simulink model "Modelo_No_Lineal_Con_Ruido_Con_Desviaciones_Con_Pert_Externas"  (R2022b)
settings: Solver=ode4  StartTime=0.0  StopTime=0.2  FixedStep=1e-6  RelTol=1e-3
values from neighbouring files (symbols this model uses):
  C_DC = 6.8e-3    (= 0.0068)    [Sistema_no_lineal_Modal.m]    (also in Sistema_no_lineal_LQR.m; PI_Lazo_V_DC.m; LQR_Sin_Integral.m; LQR_Con_Integral.m)
  control = eye(2)    [Sistema_no_lineal_Modal.m]    (also in Sistema_no_lineal_LQR.m; Sistema_control_no_lineal_LQR.m; Sistema_control_no_lineal_Modal.m)
  eta_d0_1 = ((i_q0_1*omega_1 + v_d_1/L_1 - (R_1/L_1)*i_d0_1)*(2*m_t1*L_1))/V_DC0    [Sistema_no_lineal_Modal.m]    (also in Sistema_no_lineal_LQR.m; Sistema_control_no_lineal_LQR.m; Sistema_control_no_lineal_Modal.m)
  eta_d0_2 = ((i_q0_2*omega_2 + v_d_2/L_2 - (R_2/L_2)*i_d0_2)*(2*m_t2*L_2))/V_DC0    [Sistema_no_lineal_Modal.m]    (also in Sistema_no_lineal_LQR.m; Sistema_control_no_lineal_LQR.m; Sistema_control_no_lineal_Modal.m)
  eta_q0_1 = (- i_d0_1*omega_1 - (R_1/L_1)*i_q0_1)*(2*m_t1*L_1)/V_DC0    [Sistema_no_lineal_Modal.m]    (also in Sistema_no_lineal_LQR.m; Sistema_control_no_lineal_LQR.m; Sistema_control_no_lineal_Modal.m)
  eta_q0_2 = ((- i_d0_2*omega_2 - (R_2/L_2)*i_q0_2)*(2*m_t2*L_2))/V_DC0    [Sistema_no_lineal_Modal.m]    (also in Sistema_no_lineal_LQR.m; Sistema_control_no_lineal_LQR.m; Sistema_control_no_lineal_Modal.m)
  i_d0_1 = ((3000*2)/(3*v_d_1))*1.06522    [Sistema_no_lineal_Modal.m]    (also in Sistema_no_lineal_LQR.m; PI_Lazo_V_DC.m = 14.14213562; Sistema_control_no_lineal_LQR.m; Sistema_control_no_lineal_Modal.m)
  i_d0_2 = -i_d0_1/1.06522    [Sistema_no_lineal_Modal.m]    (also in Sistema_no_lineal_LQR.m; Sistema_control_no_lineal_LQR.m; Sistema_control_no_lineal_Modal.m)
  I_p_i_d_1 = 0.02    [Sistema_no_lineal_Modal.m]    (also in Sistema_no_lineal_LQR.m; Sistema_control_no_lineal_LQR.m = 0.2; Sistema_control_no_lineal_Modal.m = 0.2)
  I_p_i_d_2 = 0.02    [Sistema_no_lineal_Modal.m]    (also in Sistema_no_lineal_LQR.m; Sistema_control_no_lineal_LQR.m = 0.2; Sistema_control_no_lineal_Modal.m = 0.2)
  I_p_i_q_1 = 0.02    [Sistema_no_lineal_Modal.m]    (also in Sistema_no_lineal_LQR.m; Sistema_control_no_lineal_LQR.m = 0.2; Sistema_control_no_lineal_Modal.m = 0.2)
  i_q0_1 = 0    [Sistema_no_lineal_Modal.m]    (also in Sistema_no_lineal_LQR.m; Sistema_control_no_lineal_LQR.m; Sistema_control_no_lineal_Modal.m)
  i_q0_2 = 0    [Sistema_no_lineal_Modal.m]    (also in Sistema_no_lineal_LQR.m; Sistema_control_no_lineal_LQR.m; Sistema_control_no_lineal_Modal.m)
  Inst_Desv_C_DC = 0.1    [Sistema_no_lineal_Modal.m]    (also in Sistema_no_lineal_LQR.m; Sistema_control_no_lineal_LQR.m; Sistema_control_no_lineal_Modal.m)
  Inst_Desv_L_1 = 0.1    [Sistema_no_lineal_Modal.m]    (also in Sistema_no_lineal_LQR.m; Sistema_control_no_lineal_LQR.m; Sistema_control_no_lineal_Modal.m)
  Inst_Desv_L_2 = 0.1    [Sistema_no_lineal_Modal.m]    (also in Sistema_no_lineal_LQR.m; Sistema_control_no_lineal_LQR.m; Sistema_control_no_lineal_Modal.m)
  Inst_Desv_R_1 = 0.1    [Sistema_no_lineal_Modal.m]    (also in Sistema_no_lineal_LQR.m; Sistema_control_no_lineal_LQR.m; Sistema_control_no_lineal_Modal.m)
  Inst_Desv_R_2 = 0.1    [Sistema_no_lineal_Modal.m]    (also in Sistema_no_lineal_LQR.m; Sistema_control_no_lineal_LQR.m; Sistema_control_no_lineal_Modal.m)
  Kc1 = Kca_place1(:, 1:2)    [Sistema_no_lineal_Modal.m]    (also in Sistema_no_lineal_LQR.m = Kca1(:, 1:2); Sistema_control_no_lineal_LQR.m = Kca1(:, 1:2); Sistema_control_no_lineal_Modal.m)
  Kc2 = Kca_place2(:, 1:2)    [Sistema_no_lineal_Modal.m]    (also in Sistema_no_lineal_LQR.m = Kca2(:, 1:2); Sistema_control_no_lineal_LQR.m = Kca2(:, 1:2); Sistema_control_no_lineal_Modal.m)
  Ki1 = -Kca_place1(:, 3:4)    [Sistema_no_lineal_Modal.m]    (also in Sistema_no_lineal_LQR.m = -Kca1(:, 3:4); Sistema_control_no_lineal_LQR.m = -Kca1(:, 3:4); Sistema_control_no_lineal_Modal.m)
  Ki2 = -Kca_place2(:, 3:4)    [Sistema_no_lineal_Modal.m]    (also in Sistema_no_lineal_LQR.m = -Kca2(:, 3:4); Sistema_control_no_lineal_LQR.m = -Kca2(:, 3:4); Sistema_control_no_lineal_Modal.m)
  L_1 = 4.1e-3    (= 0.0041)    [Sistema_no_lineal_Modal.m]    (also in Sistema_no_lineal_LQR.m; Generadores_y_tranformadas.m; LQR_Sin_Integral.m; LQR_Con_Integral.m)
  L_2 = 5.3e-3    (= 0.0053)    [Sistema_no_lineal_Modal.m]    (also in Sistema_no_lineal_LQR.m; Generadores_y_tranformadas.m; Sistema_control_no_lineal_LQR.m; Sistema_control_no_lineal_Modal.m)
  m_t1 = 5    [Sistema_no_lineal_Modal.m]    (also in Sistema_no_lineal_LQR.m; LQR_Sin_Integral.m; LQR_Con_Integral.m; Modal_Integral.m)
  m_t2 = 5    [Sistema_no_lineal_Modal.m]    (also in Sistema_no_lineal_LQR.m; Sistema_control_no_lineal_LQR.m; Sistema_control_no_lineal_Modal.m)
  omega_1 = 377    [Sistema_no_lineal_Modal.m]    (also in Sistema_no_lineal_LQR.m; LQR_Sin_Integral.m; LQR_Con_Integral.m; Modal_Integral.m)
  omega_2 = 377    [Sistema_no_lineal_Modal.m]    (also in Sistema_no_lineal_LQR.m; Sistema_control_no_lineal_LQR.m; Sistema_control_no_lineal_Modal.m)
  p_i_d_1 = 1.5    [Sistema_no_lineal_Modal.m]    (also in Sistema_no_lineal_LQR.m; Sistema_control_no_lineal_LQR.m = 2.5; Sistema_control_no_lineal_Modal.m = 2.5)
  p_i_d_2 = 1.7    [Sistema_no_lineal_Modal.m]    (also in Sistema_no_lineal_LQR.m; Sistema_control_no_lineal_LQR.m = 2.7; Sistema_control_no_lineal_Modal.m = 2.7)
  p_i_q_1 = -1.3    [Sistema_no_lineal_Modal.m]    (also in Sistema_no_lineal_LQR.m; Sistema_control_no_lineal_LQR.m = -0.5; Sistema_control_no_lineal_Modal.m = -0.5)
  Porc_Desv_C_DC = 0.05    [Sistema_no_lineal_Modal.m]    (also in Sistema_no_lineal_LQR.m; Sistema_control_no_lineal_LQR.m; Sistema_control_no_lineal_Modal.m)
  Porc_Desv_L_1 = 0.05    [Sistema_no_lineal_Modal.m]    (also in Sistema_no_lineal_LQR.m; Sistema_control_no_lineal_LQR.m; Sistema_control_no_lineal_Modal.m)
  Porc_Desv_L_2 = 0.05    [Sistema_no_lineal_Modal.m]    (also in Sistema_no_lineal_LQR.m; Sistema_control_no_lineal_LQR.m; Sistema_control_no_lineal_Modal.m)
  Porc_Desv_R_1 = 0.05    [Sistema_no_lineal_Modal.m]    (also in Sistema_no_lineal_LQR.m; Sistema_control_no_lineal_LQR.m; Sistema_control_no_lineal_Modal.m)
  Porc_Desv_R_2 = 0.05    [Sistema_no_lineal_Modal.m]    (also in Sistema_no_lineal_LQR.m; Sistema_control_no_lineal_LQR.m; Sistema_control_no_lineal_Modal.m)
  R_1 = 284e-3    (= 0.284)    [Sistema_no_lineal_Modal.m]    (also in Sistema_no_lineal_LQR.m; Generadores_y_tranformadas.m; LQR_Sin_Integral.m; LQR_Con_Integral.m)
  R_2 = 330e-3    (= 0.33)    [Sistema_no_lineal_Modal.m]    (also in Sistema_no_lineal_LQR.m; Generadores_y_tranformadas.m; Sistema_control_no_lineal_LQR.m; Sistema_control_no_lineal_Modal.m)
  tau = te    (= 0.001)    [Sistema_no_lineal_Modal.m]    (also in Sistema_no_lineal_LQR.m; IP_Lazo_P_2.m = 0.002; IP_Lazo_Q_12.m = 0.002; LQR_Sin_Integral.m = 0.002)
  v_d_1 = 100*sqrt(2)    [Sistema_no_lineal_Modal.m]    (also in Sistema_no_lineal_LQR.m; PI_Lazo_V_DC.m; LQR_Sin_Integral.m; LQR_Con_Integral.m)
  v_d_2 = 100*sqrt(2)    [Sistema_no_lineal_Modal.m]    (also in Sistema_no_lineal_LQR.m; IP_Lazo_P_2.m; Sistema_control_no_lineal_LQR.m; Sistema_control_no_lineal_Modal.m)
  V_DC0 = 500    [Sistema_no_lineal_Modal.m]    (also in Sistema_no_lineal_LQR.m; PI_Lazo_V_DC.m; LQR_Sin_Integral.m; LQR_Con_Integral.m)
  V_R_i = D_R_i^2    (= 2.5e-05)    [Sistema_no_lineal_Modal.m]    (also in Sistema_no_lineal_LQR.m; LQR_Con_Integral.m; Modal_Integral.m; Sistema_control_no_lineal_LQR.m)
  V_R_V = D_R_V^2    (= 4e-06)    [Sistema_no_lineal_Modal.m]    (also in Sistema_no_lineal_LQR.m; PI_Lazo_V_DC.m = 0.0009; Sistema_control_no_lineal_LQR.m = 0.0009; Sistema_control_no_lineal_Modal.m = 0.0009)

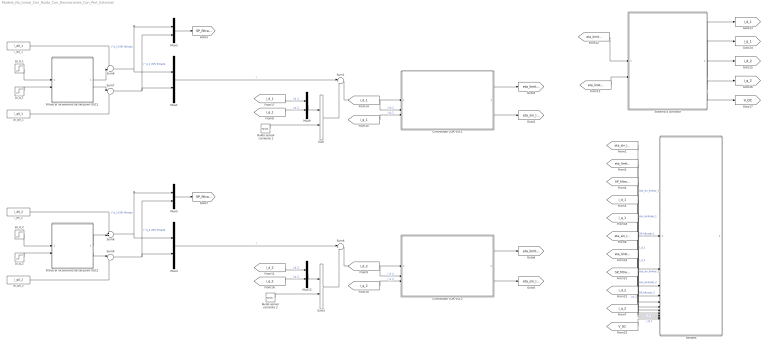
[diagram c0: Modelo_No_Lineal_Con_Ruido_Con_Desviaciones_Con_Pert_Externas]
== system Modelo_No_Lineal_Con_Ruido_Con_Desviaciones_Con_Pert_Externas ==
  Controlador LQR VSC1 : Subsystem
  Controlador LQR VSC2 : Subsystem
  Filtros al incremento de set-point VSC1 : Subsystem
  Filtros al incremento de set-point VSC2 : Subsystem
  Mux{1..2,4..5,9,12} (6 alike) : Mux  Inputs=2
  Ruido sensor corriente 1 : RandomNumber  Variance=V_R_i  SampleTime=0.001
  Ruido sensor corriente 2 : RandomNumber  Variance=V_R_i  SampleTime=0.001
  Señales : Subsystem
  Sistema a controlar : Subsystem
  Sum : Sum
  Sum1 : Sum  Inputs=|+-
  Sum2 : Sum
  Sum4 : Sum  Inputs=|+-
  Sum6 : Sum  Inputs=++|
  Sum7 : Sum  Inputs=|++
  Sum8 : Sum  Inputs=++|
  Sum9 : Sum  Inputs=|++
  i_d0_1 : Constant  Value=i_d0_1
  i_d0_2 : Constant  Value=i_d0_2
  Δi_d_1 : Step  Time=0.05  After=i_d0_1*0.05  SampleTime=0
  Δi_d_2 : Step  Time=0.05  After=i_d0_2*0.05  SampleTime=0
  Δi_q0_1 : Constant  Value=i_q0_1
  Δi_q0_2 : Constant  Value=i_q0_2
  Δi_q_1 : Step  Time=0.05  After=i_q0_1+0.5  SampleTime=0
  Δi_q_2 : Step  Time=0.05  After=i_q0_2-0.5  SampleTime=0
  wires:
  Mux2/1 -> [SP_filtrado_1]
  Δi_d_1/1 -> Filtros al incremento de set-point VSC1/1(Δi_d_1 sin filtrar)
  Δi_q_1/1 -> Filtros al incremento de set-point VSC1/2(Δi_q_1 sin filtrar)
  [eta_sin_limitar_1] -> Señales/1(eta_sin_limitar_1)  "eta_sin_limitar_1"
  [eta_limitado_1] -> Señales/2(eta_limitado_1)  "eta_limitado_1"
  [SP_filtrado_1] -> Señales/3(SP_filtrado_1)  "SP_filtrado_1"
  [i_d_1] -> Señales/4(i_d_1)  "i_d_1"
  Sum6/1 -> Mux2/1, Mux1/1  "i^d_1 (SP) filtrado"
  Sum7/1 -> Mux2/2, Mux1/2  "i^q_1 (SP) filtrado"
  Mux1/1 -> Sum1/1  "r"
  Sum9/1 -> Mux5/2, Mux4/2  "i^q_2 (SP) filtrado"
  Sum8/1 -> Mux4/1, Mux5/1  "i^d_2 (SP) filtrado"
  Mux5/1 -> [SP_filtrado_2]
  Sistema a controlar/1(i_d_1) -> [i_d_1]
  Sistema a controlar/2(i_q_1) -> [i_q_1]
  Sistema a controlar/3(i_d_2) -> [i_d_2]
  Sistema a controlar/4(i_q_2) -> [i_q_2]
  Sistema a controlar/5(V_DC) -> [V_DC]
  [eta_limitado_1] -> Sistema a controlar/1(eta limitado 1)
  [eta_limitado_2] -> Sistema a controlar/2(eta limitado 2)
  [i_d_1] -> Mux9/1  "i_d_2"
  [i_q_1] -> Mux9/2  "i_q_2"
  Mux9/1 -> Sum/1
  [i_q_1] -> Señales/5(i_q_1)  "i_q_1"
  [eta_sin_limitar_2] -> Señales/6(eta_sin_limitar_2)  "eta_sin_limitar_2"
  [eta_limitado_2] -> Señales/7(eta_limitado_2)  "eta_limitado_2"
  [SP_filtrado_2] -> Señales/8(SP_filtrado_2)  "SP_filtrado_2"
  [i_d_2] -> Señales/9(i_d_2)  "i_d_1"
  [i_q_2] -> Señales/10(i_q_2)  "i_q_1"
  [V_DC] -> Señales/11(V_DC)  "i_q_1"
  Mux12/1 -> Sum2/1
  [i_q_2] -> Mux12/2  "i_q_2"
  [i_d_2] -> Mux12/1  "i_d_2"
  Mux4/1 -> Sum4/1  "r"
  Filtros al incremento de set-point VSC1/1(Δi_d_1 filtrado) -> Sum6/2
  Filtros al incremento de set-point VSC1/2(Δi_q_1 filtrado) -> Sum7/1
  i_d0_1/1 -> Sum6/1
  Δi_q0_1/1 -> Sum7/2
  Δi_q0_2/1 -> Sum9/2
  i_d0_2/1 -> Sum8/1
  Filtros al incremento de set-point VSC2/2(Δi_q_2 filtrado) -> Sum9/1
  Filtros al incremento de set-point VSC2/1(Δi_d_2 filtrado) -> Sum8/2
  Δi_q_2/1 -> Filtros al incremento de set-point VSC2/2(Δi_q_2 sin filtrar)
  Δi_d_2/1 -> Filtros al incremento de set-point VSC2/1(Δi_d_2 sin filtrar)
  Sum1/1 -> Controlador LQR VSC1/1(e)
  [i_d_1] -> Controlador LQR VSC1/2(i_d_1)  "i_d_1"
  [i_q_1] -> Controlador LQR VSC1/3(i_q_1)  "i_q_1"
  Controlador LQR VSC1/1(eta limitado 1) -> [eta_limitado_1]
  Controlador LQR VSC1/2(eta sin limitar 1) -> [eta_sin_limitar_1]
  Sum4/1 -> Controlador LQR VSC2/1(e)
  [i_d_2] -> Controlador LQR VSC2/2(i_d_2)  "i_d_2"
  [i_q_2] -> Controlador LQR VSC2/3(i_q_2)  "i_q_2"
  Controlador LQR VSC2/1(eta limitado 2) -> [eta_limitado_2]
  Controlador LQR VSC2/2(eta sin limitar 2) -> [eta_sin_limitar_2]
  Ruido sensor corriente 1/1 -> Sum/2
  Ruido sensor corriente 2/1 -> Sum2/2
  Sum2/1 -> Sum4/2
  Sum/1 -> Sum1/2

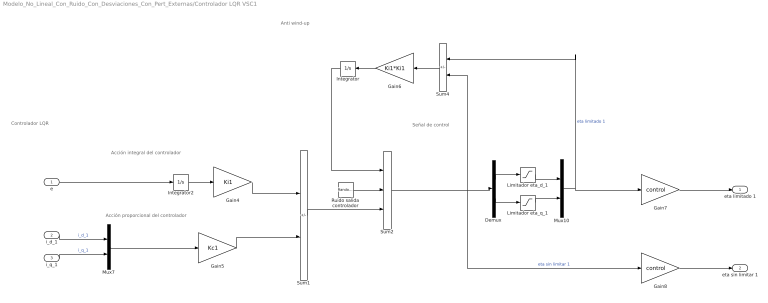
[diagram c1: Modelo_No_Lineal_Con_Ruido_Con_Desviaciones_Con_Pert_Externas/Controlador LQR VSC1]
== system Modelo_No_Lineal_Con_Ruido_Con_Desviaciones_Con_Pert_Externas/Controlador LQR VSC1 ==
  note: Anti wind-up
  note: Controlador LQR
  note: Acción proporcional del controlador
  note: Acción integral del controlador
  note: Señal de control
  e : Inport
  i_d_1 : Inport  Port=2
  i_q_1 : Inport  Port=3
  Demux : Demux  Outputs=2
  Gain4 : Gain  Gain=Ki1  Multiplication=Matrix(K*u) (u vector)
  Gain5 : Gain  Gain=Kc1  Multiplication=Matrix(K*u) (u vector)
  Gain6 : Gain  Gain=Ki1*Ki1  Multiplication=Matrix(K*u) (u vector)
  Gain7 : Gain  Gain=control  Multiplication=Matrix(K*u) (u vector)
  Gain8 : Gain  Gain=control  Multiplication=Matrix(K*u) (u vector)
  Integrator : Integrator
  Integrator2 : Integrator
  Limitador eta_d_1 : Saturate  UpperLimit=5 - eta_d0_1  LowerLimit=-5 - eta_d0_1
  Limitador eta_q_1 : Saturate  UpperLimit=5 - eta_q0_1  LowerLimit=-5 - eta_q0_1
  Mux10 : Mux  Inputs=2
  Mux7 : Mux  Inputs=2
  Ruido salida controlador : RandomNumber  Variance=V_R_V  SampleTime=0.001
  Sum1 : Sum  Inputs=+-
  Sum2 : Sum  Inputs=+++
  Sum4 : Sum  Inputs=+-
  eta limitado 1 : Outport
  eta sin limitar 1 : Outport  Port=2
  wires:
  i_q_1/1 -> Mux7/2  "i_q_1"
  Mux10/1 -> Sum4/1, Gain7/1  "eta limitado 1"
  Limitador eta_q_1/1 -> Mux10/2
  i_d_1/1 -> Mux7/1  "i_d_1"
  Limitador eta_d_1/1 -> Mux10/1
  Demux/2 -> Limitador eta_q_1/1
  Gain8/1 -> eta sin limitar 1/1
  Sum2/1 -> Gain8/1, Demux/1, Sum4/2  "eta sin limitar 1"
  Gain7/1 -> eta limitado 1/1
  Demux/1 -> Limitador eta_d_1/1
  Gain5/1 -> Sum1/2
  Gain4/1 -> Sum1/1
  Sum4/1 -> Gain6/1
  Mux7/1 -> Gain5/1
  Gain6/1 -> Integrator/1
  Sum1/1 -> Sum2/3
  Integrator2/1 -> Gain4/1
  e/1 -> Integrator2/1
  Integrator/1 -> Sum2/1
  Ruido salida controlador/1 -> Sum2/2

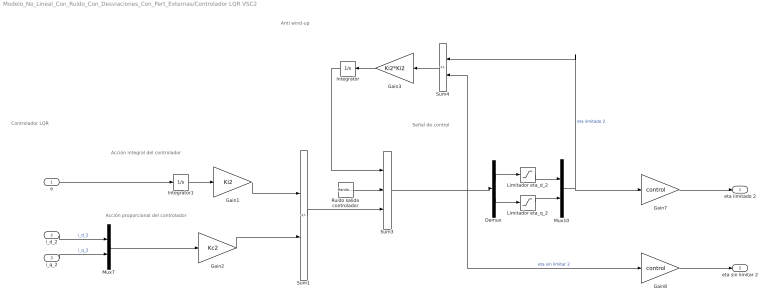
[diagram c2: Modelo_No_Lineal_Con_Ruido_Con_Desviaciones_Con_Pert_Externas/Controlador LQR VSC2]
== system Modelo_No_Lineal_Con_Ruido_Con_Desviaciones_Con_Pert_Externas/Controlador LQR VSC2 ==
  note: Señal de control
  note: Anti wind-up
  note: Acción proporcional del controlador
  note: Controlador LQR
  note: Acción integral del controlador
  e : Inport
  i_d_2 : Inport  Port=2
  i_q_2 : Inport  Port=3
  Demux : Demux  Outputs=2
  Gain1 : Gain  Gain=Ki2  Multiplication=Matrix(K*u) (u vector)
  Gain2 : Gain  Gain=Kc2  Multiplication=Matrix(K*u) (u vector)
  Gain3 : Gain  Gain=Ki2*Ki2  Multiplication=Matrix(K*u) (u vector)
  Gain7 : Gain  Gain=control  Multiplication=Matrix(K*u) (u vector)
  Gain8 : Gain  Gain=control  Multiplication=Matrix(K*u) (u vector)
  Integrator : Integrator
  Integrator1 : Integrator
  Limitador eta_d_2 : Saturate  UpperLimit=5 - eta_d0_2  LowerLimit=-5 - eta_d0_2
  Limitador eta_q_2 : Saturate  UpperLimit=5 - eta_q0_2  LowerLimit=-5 - eta_q0_2
  Mux10 : Mux  Inputs=2
  Mux7 : Mux  Inputs=2
  Ruido salida controlador : RandomNumber  Variance=V_R_V  SampleTime=0.001
  Sum1 : Sum  Inputs=+-
  Sum3 : Sum  Inputs=+++
  Sum4 : Sum  Inputs=+-
  eta limitado 2 : Outport
  eta sin limitar 2 : Outport  Port=2
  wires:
  Gain8/1 -> eta sin limitar 2/1
  Integrator/1 -> Sum3/1
  Mux7/1 -> Gain2/1
  i_d_2/1 -> Mux7/1  "i_d_2"
  Mux10/1 -> Sum4/1, Gain7/1  "eta limitado 2"
  Gain7/1 -> eta limitado 2/1
  Sum3/1 -> Gain8/1, Demux/1, Sum4/2  "eta sin limitar 2"
  i_q_2/1 -> Mux7/2  "i_q_2"
  Limitador eta_d_2/1 -> Mux10/1
  Limitador eta_q_2/1 -> Mux10/2
  Integrator1/1 -> Gain1/1
  Demux/2 -> Limitador eta_q_2/1
  Demux/1 -> Limitador eta_d_2/1
  Sum4/1 -> Gain3/1
  Gain3/1 -> Integrator/1
  Sum1/1 -> Sum3/3
  Gain1/1 -> Sum1/1
  Gain2/1 -> Sum1/2
  e/1 -> Integrator1/1
  Ruido salida controlador/1 -> Sum3/2

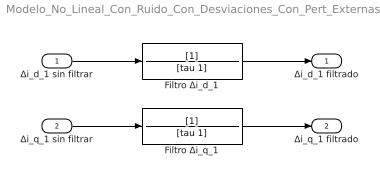
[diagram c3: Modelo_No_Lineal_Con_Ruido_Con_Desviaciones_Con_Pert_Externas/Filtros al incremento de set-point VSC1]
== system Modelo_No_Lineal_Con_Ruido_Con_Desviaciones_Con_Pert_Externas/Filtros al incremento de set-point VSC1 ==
  Δi_d_1 sin filtrar : Inport
  Δi_q_1 sin filtrar : Inport  Port=2
  Filtro Δi_d_1 : TransferFcn  Denominator=[tau 1]
  Filtro Δi_q_1 : TransferFcn  Denominator=[tau 1]
  Δi_d_1 filtrado : Outport
  Δi_q_1 filtrado : Outport  Port=2
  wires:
  Δi_q_1 sin filtrar/1 -> Filtro Δi_q_1/1
  Δi_d_1 sin filtrar/1 -> Filtro Δi_d_1/1
  Filtro Δi_d_1/1 -> Δi_d_1 filtrado/1
  Filtro Δi_q_1/1 -> Δi_q_1 filtrado/1

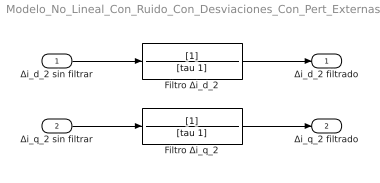
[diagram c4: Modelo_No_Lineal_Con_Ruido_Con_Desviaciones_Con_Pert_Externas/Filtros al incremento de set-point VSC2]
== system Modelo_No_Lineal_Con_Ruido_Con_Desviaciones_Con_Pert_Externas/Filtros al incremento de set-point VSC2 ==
  Δi_d_2 sin filtrar : Inport
  Δi_q_2 sin filtrar : Inport  Port=2
  Filtro Δi_d_2 : TransferFcn  Denominator=[tau 1]
  Filtro Δi_q_2 : TransferFcn  Denominator=[tau 1]
  Δi_d_2 filtrado : Outport
  Δi_q_2 filtrado : Outport  Port=2
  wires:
  Filtro Δi_q_2/1 -> Δi_q_2 filtrado/1
  Filtro Δi_d_2/1 -> Δi_d_2 filtrado/1
  Δi_d_2 sin filtrar/1 -> Filtro Δi_d_2/1
  Δi_q_2 sin filtrar/1 -> Filtro Δi_q_2/1

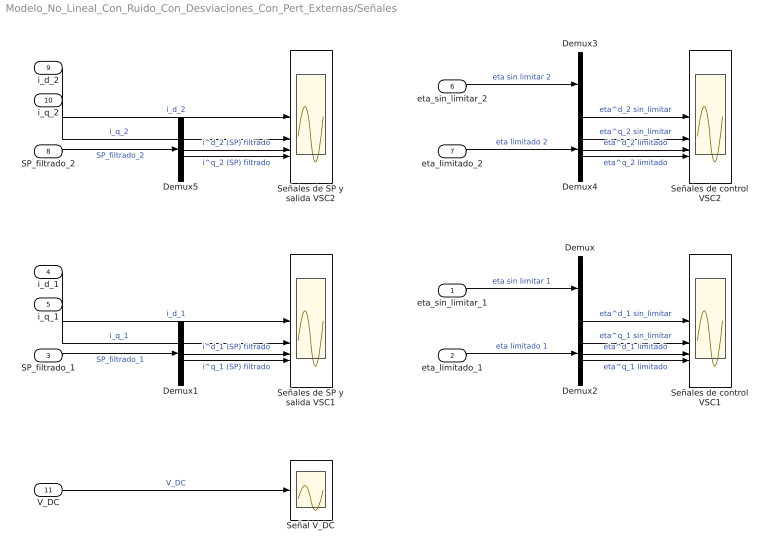
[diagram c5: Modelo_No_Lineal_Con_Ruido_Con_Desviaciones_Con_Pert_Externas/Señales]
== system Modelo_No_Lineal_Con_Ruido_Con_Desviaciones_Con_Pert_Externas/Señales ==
  eta_sin_limitar_1 : Inport
  eta_limitado_1 : Inport  Port=2
  SP_filtrado_1 : Inport  Port=3
  i_d_1 : Inport  Port=4
  i_q_1 : Inport  Port=5
  eta_sin_limitar_2 : Inport  Port=6
  eta_limitado_2 : Inport  Port=7
  SP_filtrado_2 : Inport  Port=8
  i_d_2 : Inport  Port=9
  i_q_2 : Inport  Port=10
  V_DC : Inport  Port=11
  Demux{,1..5} (6 alike) : Demux  Outputs=2
  Señal V_DC : Scope
  Señales de control VSC1 : Scope  NumInputPorts=4
  Señales de control VSC2 : Scope  NumInputPorts=4
  Señales de SP y salida VSC1 : Scope  NumInputPorts=4
  Señales de SP y salida VSC2 : Scope  NumInputPorts=4
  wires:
  i_d_1/1 -> Señales de SP y salida VSC1/1  "i_d_1"
  eta_sin_limitar_1/1 -> Demux/1  "eta sin limitar 1"
  SP_filtrado_1/1 -> Demux1/1  "SP_filtrado_1"
  eta_limitado_1/1 -> Demux2/1  "eta limitado 1"
  eta_sin_limitar_2/1 -> Demux3/1  "eta sin limitar 2"
  eta_limitado_2/1 -> Demux4/1  "eta limitado 2"
  SP_filtrado_2/1 -> Demux5/1  "SP_filtrado_2"
  i_q_1/1 -> Señales de SP y salida VSC1/2  "i_q_1"
  i_q_2/1 -> Señales de SP y salida VSC2/2  "i_q_2"
  i_d_2/1 -> Señales de SP y salida VSC2/1  "i_d_2"
  V_DC/1 -> Señal V_DC/1  "V_DC"
  Demux5/2 -> Señales de SP y salida VSC2/4  "i^q_2 (SP) filtrado"
  Demux5/1 -> Señales de SP y salida VSC2/3  "i^d_2 (SP) filtrado"
  Demux1/1 -> Señales de SP y salida VSC1/3  "i^d_1 (SP) filtrado"
  Demux1/2 -> Señales de SP y salida VSC1/4  "i^q_1 (SP) filtrado"
  Demux2/2 -> Señales de control VSC1/4  "eta^q_1 limitado"
  Demux/2 -> Señales de control VSC1/2  "eta^q_1 sin_limitar"
  Demux2/1 -> Señales de control VSC1/3  "eta^d_1 limitado"
  Demux/1 -> Señales de control VSC1/1  "eta^d_1 sin_limitar"
  Demux3/1 -> Señales de control VSC2/1  "eta^d_2 sin_limitar"
  Demux4/1 -> Señales de control VSC2/3  "eta^d_2 limitado"
  Demux3/2 -> Señales de control VSC2/2  "eta^q_2 sin_limitar"
  Demux4/2 -> Señales de control VSC2/4  "eta^q_2 limitado"

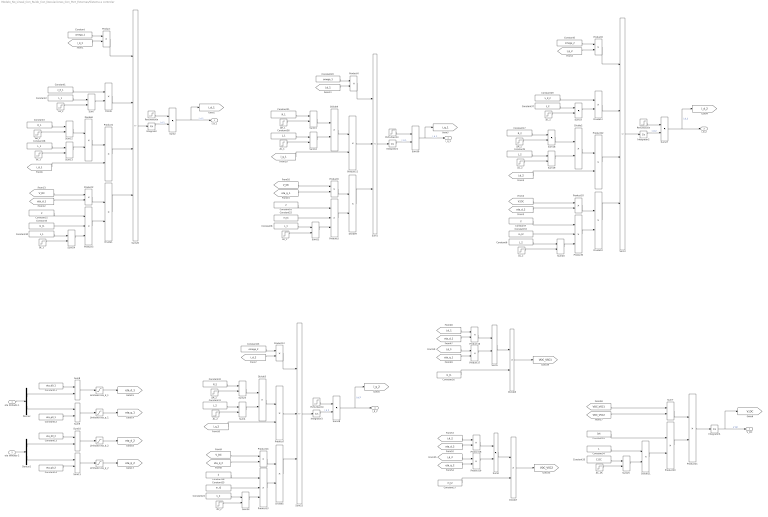
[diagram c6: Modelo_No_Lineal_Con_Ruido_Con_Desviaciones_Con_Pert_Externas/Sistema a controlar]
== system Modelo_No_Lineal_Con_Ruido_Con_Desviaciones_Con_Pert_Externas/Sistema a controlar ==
  eta limitado 1 : Inport
  eta limitado 2 : Inport  Port=2
  "  Perturbación " : Step  Time=I_p_i_d_2  After=p_i_d_2  SampleTime=0
  "  ΔL_2  " : Step  Time=Inst_Desv_L_2  After=L_2*Porc_Desv_L_2  SampleTime=0
  " Perturbación " : Step  Time=I_p_i_d_2  After=p_i_d_2  SampleTime=0
  " ΔL_1   " : Step  Time=Inst_Desv_L_1  After=L_1*Porc_Desv_L_1  SampleTime=0
  " ΔL_2  " : Step  Time=Inst_Desv_L_2  After=L_2*Porc_Desv_L_2  SampleTime=0
  Constant : Constant  Value=omega_1
  Constant1 : Constant  Value=v_d_1
  Constant11 : Constant  Value=eta_d0_1
  Constant12 : Constant  Value=eta_q0_1
  Constant13 : Constant  Value=eta_d0_2
  Constant14 : Constant  Value=eta_q0_2
  Constant{7,15..16,18} (4 alike) : Constant  Value=2
  Constant17 : Constant  Value=R_2
  Constant19 : Constant  Value=3/4
  Constant{2,8,28,30,36} (5 alike) : Constant  Value=L_1
  Constant20 : Constant  Value=omega_1
  Constant21 : Constant  Value=R_1
  Constant22 : Constant  Value=m_t1
  Constant23 : Constant  Value=omega_2
  Constant{6,9,24,31,37} (5 alike) : Constant  Value=L_2
  Constant25 : Constant  Value=m_t2
  Constant26 : Constant  Value=m_t1
  Constant27 : Constant  Value=m_t2
  Constant29 : Constant  Value=v_d_2
  Constant3 : Constant  Value=R_1
  Constant32 : Constant  Value=R_2
  Constant33 : Constant  Value=m_t2
  Constant34 : Constant
  Constant35 : Constant  Value=C_DC
  Constant4 : Constant  Value=m_t1
  Constant5 : Constant  Value=omega_2
  Demux : Demux  Outputs=2
  Demux1 : Demux  Outputs=2
  Divide{,1..12} (13 alike) : Product  Inputs=*/
  Integrator : Integrator  InitialCondition=i_d0_1
  Integrator1 : Integrator  InitialCondition=i_q0_1
  Integrator2 : Integrator  InitialCondition=i_d0_2
  Integrator3 : Integrator  InitialCondition=i_q0_2
  Integrator4 : Integrator  InitialCondition=V_DC0
  Limitador eta_d_1 : Saturate  UpperLimit=5  LowerLimit=-5
  Limitador eta_d_2 : Saturate  UpperLimit=5  LowerLimit=-5
  Limitador eta_q_1 : Saturate  UpperLimit=5  LowerLimit=-5
  Limitador eta_q_2 : Saturate  UpperLimit=5  LowerLimit=-5
  Perturbación : Step  Time=I_p_i_d_1  After=p_i_d_1  SampleTime=0
  "Perturbación " : Step  Time=I_p_i_q_1  After=p_i_q_1  SampleTime=0
  Product{,1..2,4,6..8,10..12,14,16..22} (18 alike) : Product
  Product{3,5,9,13} (4 alike) : Product  Inputs=3
  Sum{,2,4..21,23..25,27..28,30} (26 alike) : Sum
  Sum1 : Sum  Inputs=---
  Sum22 : Sum  Inputs=---
  Sum26 : Sum  Inputs=++--
  Sum3 : Sum  Inputs=++--
  ΔC_DC : Step  Time=Inst_Desv_C_DC  After=C_DC*Porc_Desv_C_DC  SampleTime=0
  ΔL_1 : Step  Time=Inst_Desv_L_1  After=L_1*Porc_Desv_L_1  SampleTime=0
  "ΔL_1 " : Step  Time=Inst_Desv_L_1  After=L_1*Porc_Desv_L_1  SampleTime=0
  "ΔL_1  " : Step  Time=Inst_Desv_L_1  After=L_1*Porc_Desv_L_1  SampleTime=0
  "ΔL_1   " : Step  Time=Inst_Desv_L_1  After=L_1*Porc_Desv_L_1  SampleTime=0
  ΔL_2 : Step  Time=Inst_Desv_L_2  After=L_2*Porc_Desv_L_2  SampleTime=0
  "ΔL_2 " : Step  Time=Inst_Desv_L_2  After=L_2*Porc_Desv_L_2  SampleTime=0
  "ΔL_2  " : Step  Time=Inst_Desv_L_2  After=L_2*Porc_Desv_L_2  SampleTime=0
  ΔR_1 : Step  Time=Inst_Desv_R_1  After=R_1*Porc_Desv_R_1  SampleTime=0
  "ΔR_1 " : Step  Time=Inst_Desv_R_1  After=R_1*Porc_Desv_R_1  SampleTime=0
  ΔR_2 : Step  Time=Inst_Desv_R_2  After=R_2*Porc_Desv_R_2  SampleTime=0
  "ΔR_2 " : Step  Time=Inst_Desv_R_2  After=R_2*Porc_Desv_R_2  SampleTime=0
  i_d_1 : Outport
  i_q_1 : Outport  Port=2
  i_d_2 : Outport  Port=3
  i_q_2 : Outport  Port=4
  V_DC : Outport  Port=5
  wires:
  Product21/1 -> Integrator4/1
  Product20/1 -> Product21/2
  Sum7/1 -> Product21/1
  Divide11/1 -> Product20/2
  Constant19/1 -> Product20/1
  [VDC_VSC2] -> Sum7/2
  [VDC_VSC1] -> Sum7/1
  Product18/1 -> Sum6/1
  Product19/1 -> Sum6/2
  [eta_d_2] -> Product18/2
  [eta_q_2] -> Product19/2
  [i_q_2] -> Product19/1
  [i_d_2] -> Product18/1
  Sum6/1 -> Divide7/1
  Constant27/1 -> Divide7/2
  Divide7/1 -> [VDC_VSC2]
  Divide6/1 -> [VDC_VSC1]
  Constant26/1 -> Divide6/2
  Sum5/1 -> Divide6/1
  [i_d_1] -> Product16/1
  [i_q_1] -> Product17/1
  [eta_q_1] -> Product17/2
  [eta_d_1] -> Product16/2
  Product17/1 -> Sum5/2
  Product16/1 -> Sum5/1
  Sum3/1 -> Integrator2/1
  Sum1/1 -> Integrator1/1
  [i_d_1] -> Product4/2
  Product4/1 -> Sum1/1
  Product11/1 -> Sum1/2
  [i_q_1] -> Product11/2
  Product6/1 -> Divide9/1
  Product5/1 -> Divide9/2
  Divide9/1 -> Sum1/3
  [V_DC] -> Product6/1
  [eta_q_1] -> Product6/2
  Constant16/1 -> Product5/1
  eta limitado 2/1 -> Demux1/1
  Constant15/1 -> Product3/1
  Constant4/1 -> Product3/2
  [eta_d_1] -> Product2/2
  [V_DC] -> Product2/1
  Divide1/1 -> Sum26/4
  Product3/1 -> Divide1/2
  Product2/1 -> Divide1/1
  [i_d_1] -> Product1/2
  Product1/1 -> Sum26/3
  Constant2/1 -> Sum/1
  Divide/1 -> Sum26/2
  Sum26/1 -> Integrator/1
  Product/1 -> Sum26/1
  [i_q_1] -> Product/2
  Integrator4/1 -> [V_DC], V_DC/1  "V_DC"
  Sum27/1 -> i_d_2/1, [i_d_2]  "i_d_2"
  Sum28/1 -> [i_q_2], i_q_2/1  "i_q_2"
  Sum30/1 -> i_q_1/1, [i_q_1]  "i_q_1"
  Constant/1 -> Product/1
  Sum2/1 -> i_d_1/1, [i_d_1]  "i_d_1"
  eta limitado 1/1 -> Demux/1
  Demux/1 -> Sum8/2
  Constant11/1 -> Sum8/1
  Sum8/1 -> Limitador eta_d_1/1
  Demux/2 -> Sum9/1
  Sum9/1 -> Limitador eta_q_1/1
  Constant12/1 -> Sum9/2
  Constant14/1 -> Sum11/2
  Demux1/2 -> Sum11/1
  Constant13/1 -> Sum10/1
  Demux1/1 -> Sum10/2
  Sum10/1 -> Limitador eta_d_2/1
  Sum11/1 -> Limitador eta_q_2/1
  Constant1/1 -> Divide/1
  Constant20/1 -> Product4/1
  Constant22/1 -> Product5/2
  Limitador eta_d_1/1 -> [eta_d_1]
  Limitador eta_q_1/1 -> [eta_q_1]
  Limitador eta_d_2/1 -> [eta_d_2]
  Limitador eta_q_2/1 -> [eta_q_2]
  Constant3/1 -> Sum12/1
  Constant28/1 -> Sum13/1
  Divide8/1 -> Product1/1
  Sum16/1 -> Divide4/2
  Constant21/1 -> Sum15/1
  Divide4/1 -> Product11/1
  Constant30/1 -> Sum14/1
  Sum21/1 -> Product5/3
  Sum20/1 -> Product9/3
  Divide2/1 -> Product22/1
  Constant9/1 -> Sum19/1
  Constant17/1 -> Sum18/1
  Constant5/1 -> Product8/1
  [i_q_2] -> Product8/2
  [i_d_2] -> Product22/2
  Product10/1 -> Divide10/1
  Product9/1 -> Divide10/2
  [V_DC] -> Product10/1
  [eta_d_2] -> Product10/2
  Constant33/1 -> Product9/2
  Constant7/1 -> Product9/1
  Product8/1 -> Sum3/1
  Divide12/1 -> Sum3/2
  Divide10/1 -> Sum3/4
  Product22/1 -> Sum3/3
  Sum24/1 -> Product13/3
  Sum23/1 -> Divide3/1
  Sum4/1 -> Divide3/2
  Constant25/1 -> Product13/2
  Constant23/1 -> Product12/1
  Constant18/1 -> Product13/1
  [eta_q_2] -> Product14/2
  [V_DC] -> Product14/1
  Divide5/1 -> Sum22/3
  Product13/1 -> Divide5/2
  Product14/1 -> Divide5/1
  [i_q_2] -> Product7/2
  Product7/1 -> Sum22/2
  Product12/1 -> Sum22/1
  [i_d_2] -> Product12/2
  ΔL_1/1 -> Sum/2
  Sum/1 -> Divide/2
  ΔR_1/1 -> Sum12/2
  "ΔL_1 "/1 -> Sum13/2
  Sum13/1 -> Divide8/2
  Sum12/1 -> Divide8/1
  "ΔL_1  "/1 -> Sum14/2
  Sum14/1 -> Product3/3
  "ΔR_1 "/1 -> Sum15/2
  Sum15/1 -> Divide4/1
  "ΔL_1   "/1 -> Sum16/2
  Constant36/1 -> Sum16/1
  ΔL_2/1 -> Sum17/2
  Sum17/1 -> Divide12/2
  Constant37/1 -> Sum17/1
  Constant29/1 -> Divide12/1
  Sum18/1 -> Divide2/1
  Sum19/1 -> Divide2/2
  "ΔL_2 "/1 -> Sum19/2
  ΔR_2/1 -> Sum18/2
  "ΔL_2  "/1 -> Sum20/2
  Constant6/1 -> Sum20/1
  Constant8/1 -> Sum21/1
  " ΔL_1   "/1 -> Sum21/2
  Divide3/1 -> Product7/1
  Constant31/1 -> Sum4/1
  " ΔL_2  "/1 -> Sum4/2
  "ΔR_2 "/1 -> Sum23/2
  Constant32/1 -> Sum23/1
  "  ΔL_2  "/1 -> Sum24/2
  Constant24/1 -> Sum24/1
  Constant34/1 -> Divide11/1
  Constant35/1 -> Sum25/1
  ΔC_DC/1 -> Sum25/2
  Sum25/1 -> Divide11/2
  Perturbación/1 -> Sum2/1
  " Perturbación "/1 -> Sum27/1
  "  Perturbación "/1 -> Sum28/1
  Sum22/1 -> Integrator3/1
  Integrator/1 -> Sum2/2  "i_d_1"
  Integrator1/1 -> Sum30/2  "i_q_1"
  "Perturbación "/1 -> Sum30/1
  Integrator2/1 -> Sum27/2  "i_d_2"
  Integrator3/1 -> Sum28/2  "i_q_2"
